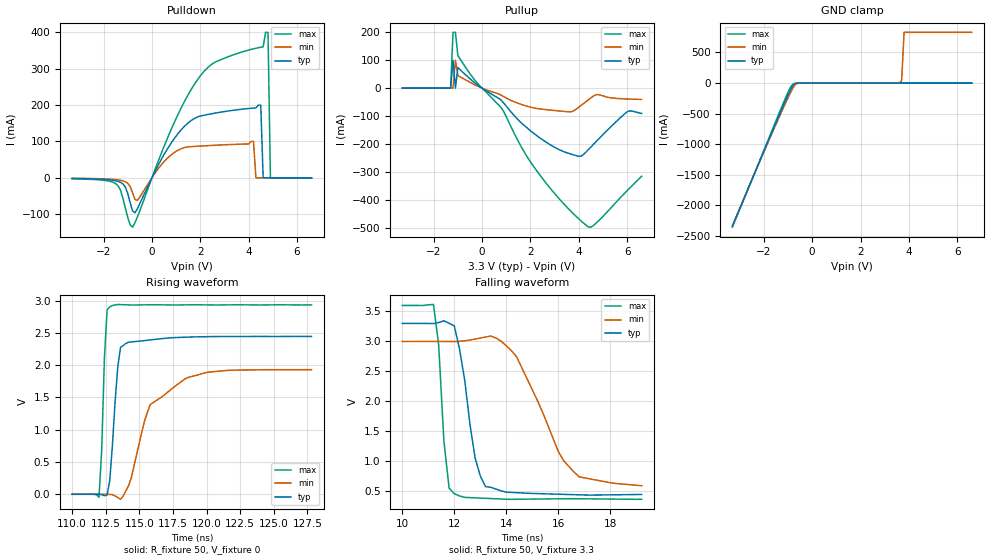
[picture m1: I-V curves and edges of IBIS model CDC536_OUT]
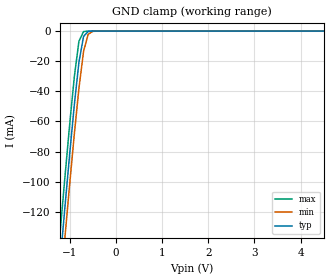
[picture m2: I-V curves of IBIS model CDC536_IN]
|   TEXAS INSTRUMENTS INCORPORATED
|   BuS Solutions Group
|   IBIS Model of CDC536
|   3.3-V PHASE LOCK LOOP Clock DRIVER WITH 3-STATE OUTPUTS
|   28-pin (DB) Package
[IBIS Ver]   2.1
[File Name]   cdc536.ibs
[File Rev]   1.0
[Date]   02/22/00
[Source]   File originated at Texas Instruments, Inc.
[Notes]   The following is an IBIS list for the CDC536.
|   - All test data contained in this file are derived from
|   hspice(tm) simulations.
|   - File created by Ramzi Ammar, BuS Solutions Applications.
[Disclaimer] Property of Texas Instruments Incorporated.  Unauthorized
   reproduction and/or distribution is strictly prohibited.
   This product is protected under copyright law.
   Created 2000, (C) Copyright 2000, Texas Instruments Inc.,
   All Rights Reserved
   UNLESS THERE IS A SIGNED, WRITTEN AGREEMENT TO THE
   CONTRARY, TEXAS INSTRUMENTS ("TI") IS PROVIDING THE IBIS
   MODELS "AS IS" AND WITHOUT ANY WARRANTY, EXPRESSED OR
   IMPLIED.  TI assumes no liability for:
   1) the accuracy of the IBIS models provided to your
   company;
   2) the proper functioning of these IBIS models in your
   design or for any resulting applications; or
   3) infringement of patents, copyrights or intellectual
   property rights resulting from your use of these IBIS
   models.
   TI provides IBIS Models as a service to our customers.
   You and your company shall not distribute, sell or give
   these models to anyone else without prior written
   permission from TI.
   TI reserves the right to make changes to our products or
   to discontinue any semiconductor product or service
   without notice, and advises our customers to obtain the
   latest version of relevant information to verify, before
   placing orders, that the information being relied on is
   current.
   Please be aware that your receipt and use of the IBIS
   information provided shall serve as acceptance of these
   terms and conditions.  If you do not accept these terms,
   you should return or destroy the IBIS models and any
   other accompanying information immediately.
[Component]   CDC536(3.3V_PLL_CLOCK_DRIVER)
[Manufacturer]  Texas Instruments, Inc.
[Package]
|   typ   min   max
R_pkg   0.043   0.038   0.048
L_pkg   1.284nH   1.088nH   1.504nH
C_pkg   0.078pF   0.068pF   0.095pF
[Pin]   signal_name   model_name
1   AVCC   POWER
2   AGND   GND
3   CLKIN   CDC536_IN
|4   SEL   CDC536_SEL
|5   NOE   CDC536_NOE
6   GND   GND
7   1Y1   CDC536_OUT
8   VCC   POWER
9   GND   GND
10   1Y2   CDC536_OUT
11   VCC   POWER
12   GND   GND
13   1Y3   CDC536_OUT
14   VCC   POWER
15   GND   GND
16   2Y3   CDC536_OUT
17   VCC   POWER
18   GND   GND
19   2Y2   CDC536_OUT
20   VCC   POWER
21   GND   GND
22   2Y1   CDC536_OUT
23   VCC   POWER
|24   NCLR   CDC536_CLR
|25   TEST   CDC536_TEST
26   FBIN   CDC536_IN
27   AGND   GND
28   AVCC   POWER
| Models and submodels in the file (2): CDC536_OUT (3-state), CDC536_IN (Input)
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|   Model CDC536_OUT
[Model]   CDC536_OUT
Model_type   3-state
Polarity   Inverting
Enable   Active-Low
Vmeas = 1.5V   |Vref for timing measurements.
Cref = 30pF   |load capacitance for timing spec.
Rref = 500   |500 Ohm to GND.
Vref = 0   |Timing specification test load voltage; GND
|   typ   min   max
C_comp   6pF   NA   9pF
[Voltage range]   3.3   3.0   3.6
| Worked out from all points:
|   slope of the pulldown table from 0 to 0.495 V, typ, clamps not added: 7.83 ohm
|   slope of the pullup table from 0 to 0.495 V, typ, clamps not added: 18.5 ohm
|   GND clamp passes 1 mA (typ) near -0.61 V on its own axis
|   rising waveform, R_fixture 50, V_fixture 0: 20-80 % time 493ps typ, 2.34ns min, 293ps max; typ from 0 V to 2.45 V
|   falling waveform, R_fixture 50, V_fixture 3.3: 20-80 % time 570ps typ, 1.48ns min, 287ps max; typ from 3.3 V to 0.446 V
| Notes: (1) Vtable = Vcc - Voutput
|   (2) Pullup data includes the effects of the ESD
|   clamping circuitry
[Pullup]
|   50C:3.3V:   100C:3V:weak   0C:3.6V:strong
|   Voltage   I(typ)   I(min)   I(max)
-3.3V     0A         0A         0A
-1.3V     0A         0A         0A
-1.2V     100mA      0A         200mA
-1.1V     0A         100mA      200mA
-1V       73.8mA     44.9mA     116.3mA
800mV     -43.8mA    -25.81mA   -70.92mA
1.7V      -130.4mA   -60.57mA   -222.3mA
3.3V      -224.6mA   -82.62mA   -407.1mA
4.3V      -229.2mA   -48.23mA   -491mA
4.6V      -202.2mA   -28.7mA    -492.5mA
6V        -84.7mA    -38.9mA    -367.4mA
6.6V      -90.7mA    -40.5mA    -315.7mA
[Pulldown]
|   50C:3.3V:   100C:3V:weak   0C:3.6V:strong
|   Voltage   I(typ)   I(min)   I(max)
-3.3V     -2mA       -1.4mA     -2.8mA
-1.5V     -8.252mA   -4.941mA   -15.98mA
-800mV    -90.82mA   -41.17mA   -135.8mA
2V        169.8mA    87.2mA     280.1mA
4.2V      191.7mA    100mA      354.6mA
4.3V      192.3mA    0A         356.1mA
4.5V      200mA      0A         359mA
4.6V      0A         0A         360.2mA
4.7V      0A         0A         400mA
4.8V      0A         0A         400mA
4.9V      0A         0A         0A
6.6V      0A         0A         0A
[GND Clamp]
|   50C:3.3V:   100C:3V:weak   0C:3.6V:strong
|   Voltage   I(typ)   I(min)   I(max)
-3.3V     -2.34A     -2.341A    -2.359A
-2.2V     -1.309A    -1.311A    -1.298A
-1.2V     -377.1mA   -413.9mA   -334.4mA
-900mV    -115.6mA   -161mA     -71.19mA
-800mV    -44.39mA   -85.93mA   -18.17mA
-700mV    -6.053mA   -27.1mA    -6.046mA
-600mV    -489uA     -2.803mA   -3.031mA
-500mV    -5.392uA   -141.2uA   -645.5uA
3.6V      3.398nA    1.65mA     1.451nA
3.7V      70.04nA    37mA       1.511nA
3.8V      2.486uA    829.4mA    1.572nA
6.6V      2.486uA    829.4mA    1.572nA
[ramp]
| variable   typ   min   max
dV/dt_r   1.4822E+00/4.7010E-10  1.2097E+00/2.3179E-09  1.7916E+00/2.5377E-10
dV/dt_f   1.7451E+00/5.7879E-10  1.5191E+00/1.5206E-09  1.9960E+00/2.6619E-10
[Rising Waveform]
R_fixture = 50
V_fixture = 0
|   50C:3.3V:   100C:3V:weak   0C:3.6V:strong
|   Time   V(typ)   V(min)   V(max)
110ns     -105.8uV   -131.4uV   -207.3uV
112ns     787.2uV    -59.3uV    -44.96mV
112.2ns   -6.04mV    158.3uV    692.6mV
112.6ns   -14.08mV   1.227mV    2.859V
112.8ns   217.2mV    -2.473mV   2.906V
113.4ns   1.981V     -52.64mV   2.941V
114ns     2.337V     54.52mV    2.936V
115.8ns   2.392V     1.39V      2.937V
118.4ns   2.434V     1.788V     2.935V
127.8ns   2.446V     1.931V     2.935V
[Falling Waveform]
R_fixture = 50
V_fixture = 3.3
V_fixture_min = 3
V_fixture_max = 3.6
|   50C:3.3V:   100C:3V:weak   0C:3.6V:strong
|   Time   V(typ)   V(min)   V(max)
10ns      3.3V       3V         3.6V
11.2ns    3.298V     3V         3.616V
11.4ns    3.315V     2.999V     2.942V
11.8ns    3.303V     2.998V     552.3mV
12ns      3.26V      2.998V     459.8mV
12.8ns    1.055V     3.039V     389.8mV
13.2ns    576.2mV    3.073V     382mV
14.4ns    476.2mV    2.739V     366.2mV
16.6ns    443.3mV    820.7mV    375.6mV
19.2ns    446.4mV    592.1mV    366mV
|   Model CDC536_IN
[Model]   CDC536_IN
Model_type   Input
Polarity   Inverting
Vinl = 0.8V
Vinh = 2.0V
|   typ   min   max
C_comp   4pF   NA   6pF
[Voltage Range]   3.3   3.0   3.6
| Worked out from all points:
|   GND clamp passes 1 mA (typ) near -0.62 V on its own axis
[GND Clamp]
|   50C:3.3V:   100C:3V:weak   0C:3.6V:strong
|   Voltage   I(typ)   I(min)   I(max)
-3.3V     -930.1mA   -948.5mA   -912.1mA
-1.3V     -186.7mA   -206.8mA   -166.9mA
-1.2V     -151mA     -171.1mA   -131.1mA
-1.1V     -115.8mA   -136mA     -95.9mA
-1V       -81.58mA   -101.6mA   -61.88mA
-900mV    -49.1mA    -68.51mA   -30.42mA
-800mV    -20.66mA   -37.98mA   -6.772mA
-700mV    -3.548mA   -13.49mA   -336.8uA
-600mV    -234.9uA   -2.144mA   -6.074uA
-500mV    -7.663uA   -188.1uA   -91.14nA
6.6V      4.604nA    4.949nA    4.671nA
